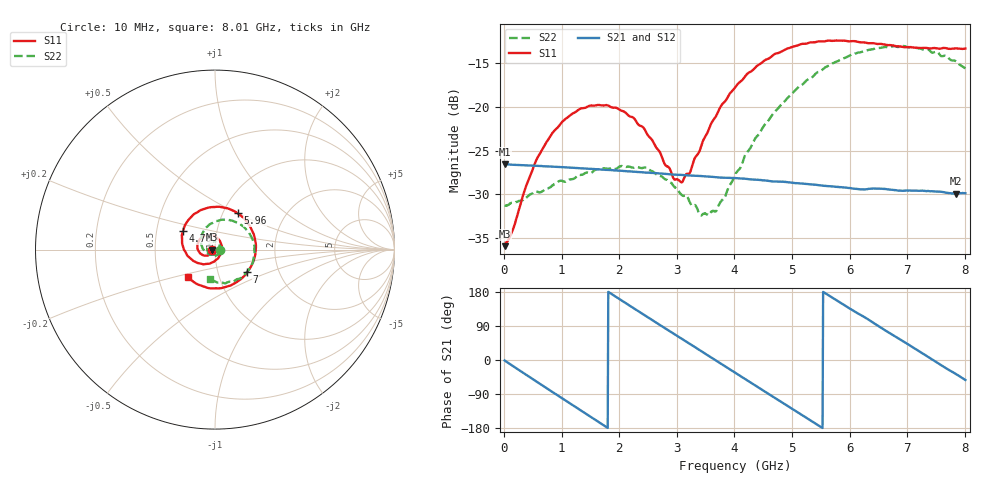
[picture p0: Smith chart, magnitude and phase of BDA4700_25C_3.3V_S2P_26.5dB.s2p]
!Agilent Technologies,E5071B,MY42404982,A.09.10
!Date: Mon Oct 20 18:14:12 2025
!Data & Calibration Information:
!Freq	S11:SOLT2(ON)	S21:SOLT2(ON)	S12:SOLT2(ON)	S22:SOLT2(ON)
# Hz S RI R 50
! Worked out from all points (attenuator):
!   801 points, 10 MHz to 8.01 GHz, reference 50 ohm
!   highest |S21| = -26.55 dB at 10 MHz (marker M1); lowest = -29.9 dB at 7.84 GHz (marker M2)
!   lowest |S11| = -36.0 dB at 10 MHz (marker M3), VSWR 1.03, Z = 48.4 - j0.105 ohm
!   |S11| at or under -10 dB: start of sweep to end of sweep
!   |S22| runs from -32.4 to -13.0 dB; largest |S21 - S12| = 0.00059
!   S11 on the Smith chart (normalised r, x): 10 MHz: 0.97, -0.00; 4.79 GHz: 0.68, +0.15; 5.96 GHz: 1.17, +0.50; 7 GHz: 1.38, -0.37; 8.01 GHz: 0.71, -0.23
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1e7  -0.0159 -0.00109  0.047 -0.000996  0.047 -0.00103  0.0272 -0.00086
1.5e8  -0.0171 -0.00988  0.0449 -0.0125  0.0449 -0.0124  0.0273 -0.00737
6e8  -0.0406 -0.0333  0.0226 -0.04  0.0226 -0.0399  0.0132 -0.0296
1.01e9  -0.0785 -0.0244  -0.00883 -0.0443  -0.00878 -0.0443  -0.0152 -0.0345
1.35e9  -0.098 0.00707  -0.0314 -0.0315  -0.0314 -0.0315  -0.0365 -0.0182
2.08e9  -0.0502 0.0797  -0.0384 0.0193  -0.0384 0.0193  -0.0302 0.0338
2.42e9  -0.00281 0.0761  -0.0213 0.0365  -0.0212 0.0364  -0.0051 0.0445
2.68e9  0.0263 0.05  -0.00359 0.0415  -0.00371 0.0414  0.0129 0.0384
2.95e9  0.0374 0.0101  0.0147 0.0382  0.0147 0.0382  0.0257 0.0238
3.09e9  0.0349 -0.0123  0.0232 0.0335  0.0229 0.0336  0.0285 0.0127
3.41e9  0.00516 -0.0574  0.0365 0.0168  0.0365 0.0169  0.0213 -0.011
3.55e9  -0.0166 -0.0716  0.0391 0.00776  0.0391 0.00767  0.0131 -0.0202
3.7e9  -0.0453 -0.079  0.0395 -0.00219  0.0395 -0.0023  0.000327 -0.026
4.01e9  -0.1094 -0.0685  0.0328 -0.0214  0.0328 -0.0212  -0.0311 -0.0261
4.79e9  -0.1782 0.1023  -0.0118 -0.0354  -0.0115 -0.0355  -0.0779 0.0643
5.35e9  -0.0685 0.2239  -0.0342 -0.0109  -0.0342 -0.0111  -0.0159 0.1469
5.96e9  0.1261 0.2023  -0.0263 0.0222  -0.0264 0.022  0.1217 0.1511
6.68e9  0.225 -0.0197  0.0103 0.032  0.0103 0.0321  0.2195 0.000301
7e9  0.1799 -0.1266  0.0243 0.0225  0.0245 0.0223  0.2033 -0.0851
7.45e9  0.0409 -0.2133  0.0329 -9.92e-05  0.0329 -0.000132  0.1131 -0.1707
7.84e9  -0.0997 -0.1918  0.0257 -0.0189  0.0257 -0.0191  0.0117 -0.1828
8.01e9  -0.1502 -0.1554  0.0194 -0.0255  0.0195 -0.0255  -0.0302 -0.1634
